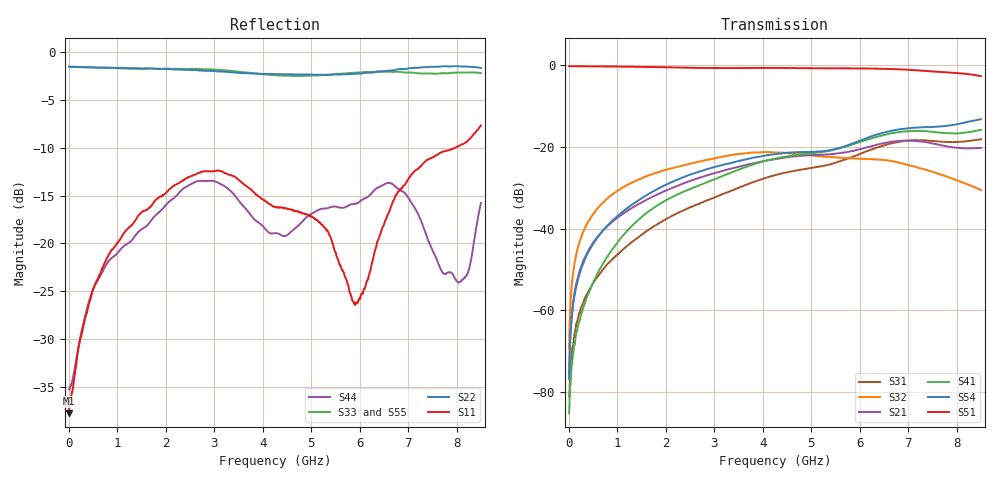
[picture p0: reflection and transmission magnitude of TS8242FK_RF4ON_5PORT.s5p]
! Created with skrf (http://scikit-rf.org).
# Hz S RI R 50.0
!freq ReS11 ImS11 ReS12 ImS12 ReS13 ImS13
! ReS14 ImS14 ReS15 ImS15
! ReS21 ImS21 ReS22 ImS22 ReS23 ImS23
! ReS24 ImS24 ReS25 ImS25
! ReS31 ImS31 ReS32 ImS32 ReS33 ImS33
! ReS34 ImS34 ReS35 ImS35
! ReS41 ImS41 ReS42 ImS42 ReS43 ImS43
! ReS44 ImS44 ReS45 ImS45
! ReS51 ImS51 ReS52 ImS52 ReS53 ImS53
! ReS54 ImS54 ReS55 ImS55
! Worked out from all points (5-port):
!   1601 points, 10 MHz to 8.5 GHz, reference 50 ohm
!   strongest paths, dB at 10 MHz, 2.132 GHz, 4.255 GHz, 6.378 GHz, 8.5 GHz:
!     S51: -0.2, -0.5, -0.6, -0.8, -2.6
!     S54: -76.9, -28.6, -21.8, -16.9, -13.2
!     S41: -85.3, -32.3, -22.9, -17.4, -15.8
!     S21: -75.4, -30.0, -23.0, -19.4, -20.2
!     S32: -69.4, -25.2, -21.4, -23.1, -30.6
!     S31: -81.1, -36.9, -26.9, -20.1, -18.1
!   lowest |S11| = -37.8 dB at 10 MHz (marker M1), VSWR 1.03, Z = 51.3 + j0.311 ohm
!   |S11| at or under -10 dB: start of sweep to 7.971 GHz
